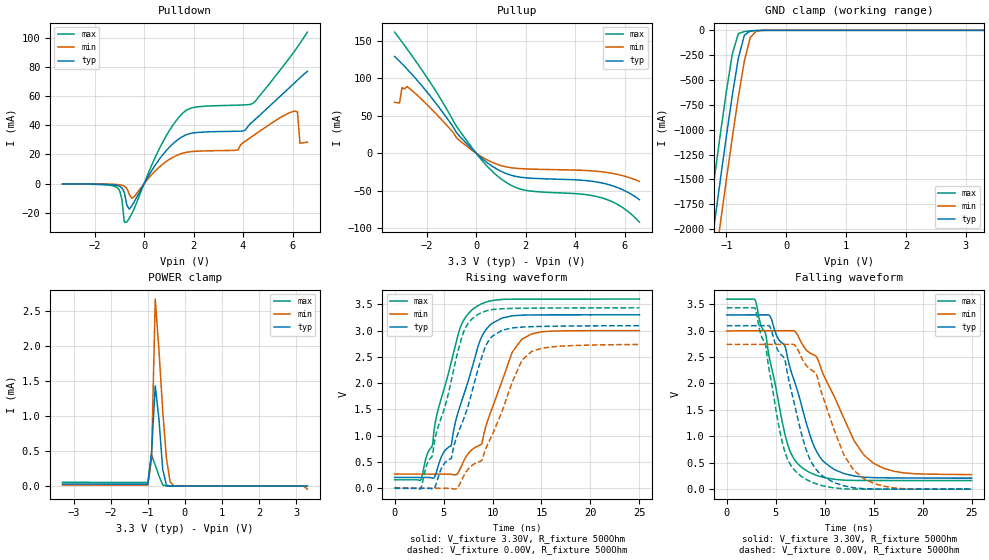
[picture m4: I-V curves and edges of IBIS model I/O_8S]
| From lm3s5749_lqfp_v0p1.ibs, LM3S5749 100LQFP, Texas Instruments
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[Model]   I/O_8S
Model_type   I/O
Vinl = 1.26
Vinh = 2.04
Vmeas = 1.65
| variable   typ   min   max
C_comp   9.739pF   9.739pF   9.803pF
[Model Spec]
Vinh+   1.91   1.78   2.04
Vinh-   1.90   1.76   2.03
Vinl+   1.40   1.27   1.54
Vinl-   1.39   1.26   1.53
| variable   typ   min   max
[Temperature Range]  25   85   -40
[Voltage Range]   3.3V   3.0V   3.6V
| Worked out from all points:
|   slope of the pulldown table from 0 to 0.495 V, typ, clamps not added: 35.8 ohm
|   slope of the pullup table from 0 to 0.495 V, typ, clamps not added: 35.8 ohm
|   GND clamp passes 1 mA (typ) near -0.48 V on its own axis
|   POWER clamp passes 1 mA (typ) near -0.71 V on its own axis
|   falling waveform, V_fixture 3.30V, R_fixture 500Ohm: 20-80 % time 2.89ns typ, 4.05ns min, 2.22ns max; typ from 3.3 V to 0.209 V
|   rising waveform, V_fixture 3.30V, R_fixture 500Ohm: 20-80 % time 2.69ns typ, 3.1ns min, 2.58ns max; typ from 0.208 V to 3.3 V
|   falling waveform, V_fixture 0.00V, R_fixture 500Ohm: 20-80 % time 2.49ns typ, 3.21ns min, 2.03ns max; typ from 3.09 V to 0 V
|   rising waveform, V_fixture 0.00V, R_fixture 500Ohm: 20-80 % time 3.02ns typ, 3.46ns min, 2.75ns max; typ from 0.001 V to 3.09 V
[Pulldown]
|  Voltage   I(typ)   I(min)   I(max)
-3.3V     -256.6uA   -145.6uA   -364.5uA
-1.1V     -1.273mA   -587.5uA   -2.567mA
-700mV    -14.71mA   -3.215mA   -26.33mA
-500mV    -15.26mA   -10mA      -20.66mA
600mV     16.36mA    11.13mA    23.41mA
1.5V      31.68mA    20.52mA    47.2mA
3.8V      35.88mA    23.15mA    53.74mA
4.4V      42.6mA     32.69mA    54.98mA
6.1V      69.26mA    49.6mA     91.12mA
6.2V      70.84mA    49.17mA    93.51mA
6.3V      72.42mA    27.66mA    95.98mA
6.6V      76.89mA    28.41mA    103.8mA
[Pullup]
|  Voltage   I(typ)   I(min)   I(max)
-3.3V     129.3mA    68.2mA     161.9mA
-3.1V     122.9mA    67.41mA    153.1mA
-3V       119.6mA    87.83mA    148.7mA
-2.8V     112.7mA    89.21mA    139.6mA
-1.8V     73.98mA    58.72mA    91.66mA
-700mV    23.83mA    17.72mA    31.29mA
300mV     -8.845mA   -6.303mA   -12.15mA
1V        -23.99mA   -16.37mA   -34.1mA
2V        -32.73mA   -20.87mA   -49.46mA
5.1V      -39.81mA   -24.88mA   -59.77mA
5.9V      -48.4mA    -29.75mA   -72.06mA
6.6V      -62.06mA   -37.61mA   -92.08mA
[GND Clamp]
|  Voltage   I(typ)   I(min)   I(max)
-3.3V     -11.73A    -12.14A    -11.32A
-1.4V     -2.85A     -3.29A     -2.391A
-1.3V     -2.393A    -2.835A    -1.933A
-1.2V     -1.942A    -2.383A    -1.481A
-1.1V     -1.496A    -1.937A    -1.038A
-1V       -1.061A    -1.498A    -612.1mA
-900mV    -646.5mA   -1.071A    -233.9mA
-800mV    -278.2mA   -665.9mA   -32.18mA
-700mV    -49.12mA   -307.7mA   -12.49mA
-600mV    -5.764mA   -70.86mA   -6.504mA
-500mV    -1.206mA   -8.171mA   -2.256mA
3.3V      2.312nA    3.21uA     471pA
[POWER Clamp]
|  Voltage   I(typ)   I(min)   I(max)
-3.3V     29.71uA    15.87uA    54.94uA
-1V       27.67uA    14.78uA    51.22uA
-900mV    475.3uA    385.2uA    446.8uA
-800mV    1.43mA     2.664mA    297.3uA
-700mV    950.8uA    1.937mA    147.8uA
-600mV    244.5uA    1.079mA    15.75uA
-500mV    13.05uA    399.9uA    1.307uA
-400mV    328.8nA    62.11uA    58.57nA
-300mV    10.28nA    3.21uA     1.749nA
3.1V      1.297nA    -118nA     134.9pA
3.2V      1.2nA      -2.426uA   122pA
3.3V      -118pA     -43.75uA   108.5pA
[Ramp]
| variable   typ   min   max
dV/dt_f   1.85/2.89n   1.63/4.05n   2.06/2.22n
dV/dt_r   1.85/3.02n   1.63/3.46n   2.06/2.75n
R_load = 500Ohm
[Falling Waveform]
V_fixture = 3.30V
V_fixture_min = 3.00V
V_fixture_max = 3.60V
R_fixture = 500Ohm
|   Time   V(typ)   V(min)   V(max)
0s        3.297V     2.993V     3.597V
2.9ns     3.298V     2.998V     3.588V
4.4ns     3.285V     2.998V     2.45V
6.2ns     2.507V     2.999V     863.5mV
7.8ns     1.474V     2.717V     393.5mV
8.9ns     822.8mV    2.539V     281.5mV
10ns      504.1mV    2.115V     218.2mV
13ns      250.1mV    920.3mV    165.8mV
15ns      218mV      489.3mV    164.4mV
25ns      208.5mV    275.7mV    162.4mV
[Rising Waveform]
V_fixture = 3.30V
V_fixture_min = 3.00V
V_fixture_max = 3.60V
R_fixture = 500Ohm
|   Time   V(typ)   V(min)   V(max)
0s        207.7mV    271.8mV    162.2mV
2.7ns     207.5mV    270.7mV    165.9mV
4.1ns     223mV      270.3mV    1.19V
5.8ns     823.8mV    267.1mV    2.412V
6.6ns     1.515V     332.8mV    2.996V
8.1ns     2.416V     762.7mV    3.421V
8.9ns     2.882V     848.2mV    3.509V
9.7ns     3.095V     1.392V     3.56V
13ns      3.293V     2.836V     3.597V
25ns      3.299V     2.999V     3.598V
[Falling Waveform]
V_fixture = 0.00V
V_fixture_min = 0.00V
V_fixture_max = 0.00V
R_fixture = 500Ohm
|   Time   V(typ)   V(min)   V(max)
0s        3.093V     2.739V     3.433V
2.9ns     3.093V     2.74V      3.423V
4ns       3.094V     2.74V      2.703V
4.4ns     3.079V     2.74V      2.187V
5.8ns     2.5V       2.741V     798.4mV
7.6ns     1.077V     2.508V     246.9mV
9.6ns     282mV      1.881V     74.67mV
12ns      61.67mV    635.6mV    6.05mV
14ns      8.398mV    200.8mV    317.7uV
25ns      42.17uV    193.1uV    23.99uV
[Rising Waveform]
V_fixture = 0.00V
V_fixture_min = 0.00V
V_fixture_max = 0.00V
R_fixture = 500Ohm
|   Time   V(typ)   V(min)   V(max)
0s        982.1uV    13.53mV    202.2uV
2.7ns     218.5uV    1.482mV    4.716mV
4ns       -9.375mV   1.191mV    805.7mV
5.8ns     575.1mV    -2.064mV   2.059V
7ns       1.294V     213.3mV    2.95V
8.2ns     2.045V     470mV      3.267V
10ns      2.895V     1.028V     3.399V
13ns      3.066V     2.434V     3.424V
14ns      3.074V     2.603V     3.426V
25ns      3.092V     2.735V     3.432V
